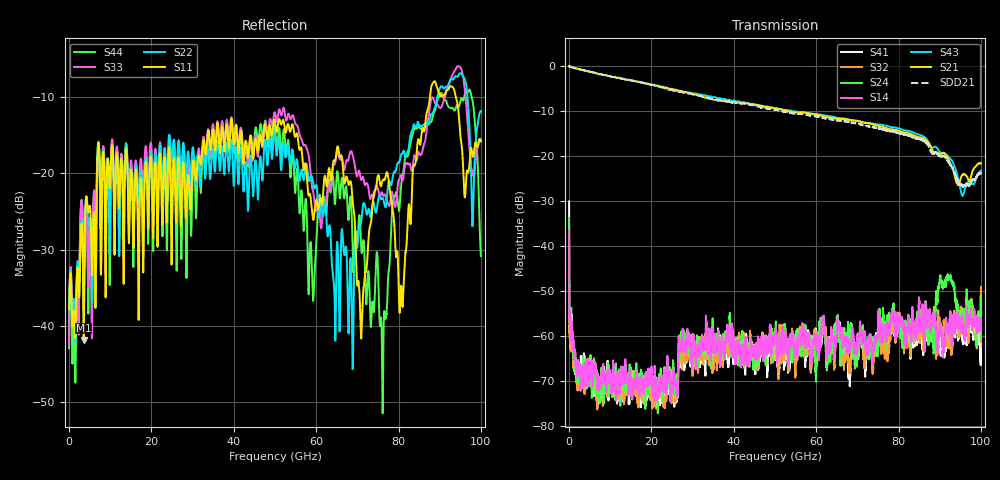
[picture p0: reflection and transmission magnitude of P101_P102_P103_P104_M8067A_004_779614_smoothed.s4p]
!Keysight Technologies PLTS 2021(64 bit), Build 20210202.1
!S11 smoothed in format LOGMAG, average points = 21
!S12 smoothed in format LOGMAG, average points = 21
!S13 smoothed in format LOGMAG, average points = 21
!S14 smoothed in format LOGMAG, average points = 21
!S21 smoothed in format LOGMAG, average points = 21
!S22 smoothed in format LOGMAG, average points = 21
!S23 smoothed in format LOGMAG, average points = 21
!S24 smoothed in format LOGMAG, average points = 21
!S31 smoothed in format LOGMAG, average points = 21
!S32 smoothed in format LOGMAG, average points = 21
!S33 smoothed in format LOGMAG, average points = 21
!S34 smoothed in format LOGMAG, average points = 21
!S41 smoothed in format LOGMAG, average points = 21
!S42 smoothed in format LOGMAG, average points = 21
!S43 smoothed in format LOGMAG, average points = 21
!S44 smoothed in format LOGMAG, average points = 21
!$DUT_CFG_DESC: Default 4-Port Configuration
!$NUMBER_PORTS: 4
!$DIFF_PORT_MAP: 1|2P|2|2P|0|UC|0|UC|
!$PORT_MAP: 1|1|<<<<<<|2|2|>>>>>>|3|3|<<<<<<|4|4|>>>>>>|
!Date: Monday, December 04, 2023, 05:51:05
!S4P File: Measurements: <S11,S12,S13,S14>,
!<S21,S22,S23,S24>,
!<S31,S32,S33,S34>,
!<S41,S42,S43,S44>:
# MHz S  RI  R 50
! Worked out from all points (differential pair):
!   10000 points, 10 MHz to 100 GHz, reference 50 ohm
!   strongest paths, dB at 10 MHz, 25.01 GHz, 50.01 GHz, 75.01 GHz, 100 GHz:
!     S21: -0.1, -5.2, -9.5, -13.4, -21.7
!     S43: -0.2, -5.4, -9.5, -13.1, -23.3
!     S14: -36.7, -71.9, -60.8, -58.5, -58.3
!     S24: -33.9, -70.9, -60.7, -61.4, -60.5
!     S32: -40.3, -71.0, -63.3, -62.8, -49.1
!     S41: -30.2, -73.9, -64.8, -60.4, -57.8
!   taken as a pair (ports 1,3 in; 2,4 out), SDD21 dB: -0.1, -5.4, -9.8, -13.9, -23.8
!   lowest |S11| = -41.9 dB at 3.55 GHz (marker M1), VSWR 1.02, Z = 50.5 + j0.644 ohm
!   |S11| at or under -10 dB: start of sweep to 87.62 GHz; 93.92 GHz to end of sweep
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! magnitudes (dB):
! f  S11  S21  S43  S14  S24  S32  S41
! 10 MHz  -37.9  -0.1  -0.2  -36.7  -33.9  -40.3  -30.2
! 3.55 GHz  -41.9  -1.0  -1.0  -66.8  -68.8  -70.2  -68.0
! 47.6 GHz  -13.6  -9.1  -9.3  -60.9  -62.2  -65.0  -63.1
! 70.95 GHz  -41.7  -12.5  -12.5  -59.2  -60.2  -60.2  -60.0
! 75.91 GHz  -21.4  -13.6  -13.1  -59.5  -59.4  -62.6  -57.5
! 96.89 GHz  -19.8  -25.2  -25.9  -57.9  -57.8  -60.4  -58.5
! 100 GHz  -15.8  -21.7  -23.3  -58.3  -60.5  -49.1  -57.8
